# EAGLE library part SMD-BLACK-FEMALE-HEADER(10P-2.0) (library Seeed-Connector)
320030097
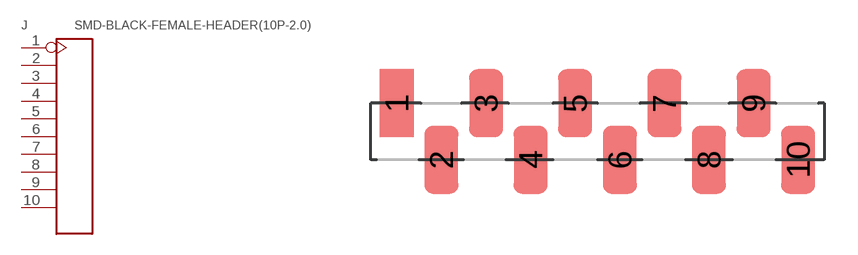
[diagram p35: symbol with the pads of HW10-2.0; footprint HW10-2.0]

Designator prefix J

## SMD-BLACK-FEMALE-HEADER(10P-2.0)-2-SMD (VALUE: 10P-SMD-2.0)  [HW10-2.0]
1  1
2  2
3  3
4  4
5  5
6  6
7  7
8  8
9  9
10  10

## Footprint HW10-2.0 (pad centres in mm)
smd 1.524 x 3.048: 1 -9,1.27; 2 -7,-1.27; 3 -5,1.27; 4 -3,-1.27; 5 -1,1.27; 6 1,-1.27; 7 3,1.27; 8 5,-1.27; 9 7,1.27; 10 9,-1.27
